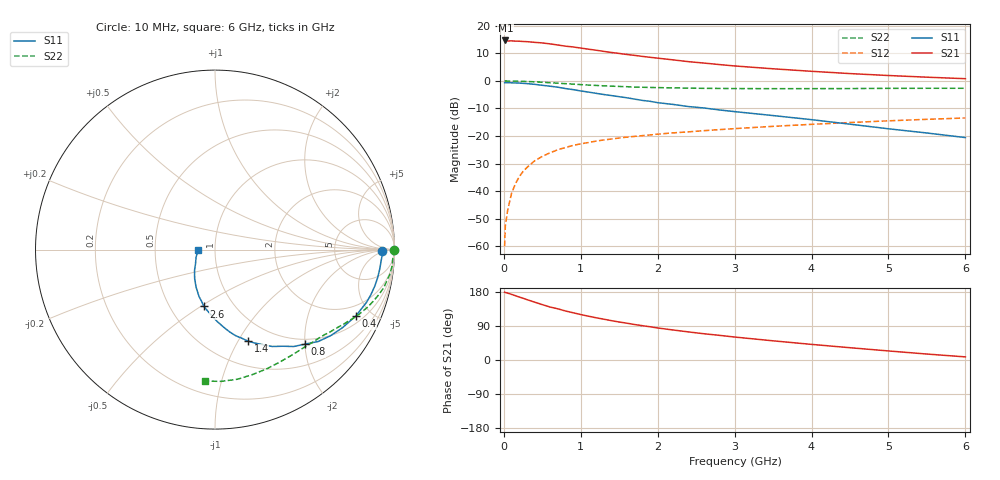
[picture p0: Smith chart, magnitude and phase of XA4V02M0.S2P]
! SIEMENS Discrete & RF Semiconductors
! BFY180
! Si NPN RF Bipolar Junction Transistor in MICRO-X
! VCE = 4 V  IC = 2 mA
! Common Emitter S-Parameters:  May  1997
# GHz  S  MA  R  50
!  f  S11  S21  S12  S22
! GHz  MAG  ANG  MAG  ANG  MAG  ANG  MAG  ANG
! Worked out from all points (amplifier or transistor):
!   36 points, 10 MHz to 6 GHz, reference 50 ohm
!   highest |S21| = 14.7 dB at 20 MHz (marker M1)
!   |S21| within 3 dB of that: start of sweep to 1.059 GHz
!   unconditionally stable (mu >= 1): 2.881 GHz to end of sweep
!   at 250 MHz: K = 0.13, MSG = 23.6 dB, |S12| = -32.9 dB
!   at 1.4 GHz: K = 0.67, MSG = 15.7 dB, |S12| = -21.1 dB
!   at 6 GHz: K = 1.06, MAG = 5.6 dB, |S12| = -13.5 dB
!   S11 on the Smith chart (normalised r, x): 10 MHz: 26, -4; 400 MHz: 1.35, -4.03; 800 MHz: 0.90, -2.00; 1.4 GHz: 0.76, -1.10; 2.6 GHz: 0.73, -0.52; 6 GHz: 0.83, -0.00
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0.01  0.9286 -0.6  5.365 179.0  0.001 88.0  0.9949 -0.2
0.02  0.933 -1.5  5.428 178.1  0.0024 83.0  0.9999 -0.7
0.05  0.9292 -3.1  5.312 176.6  0.0045 87.0  0.9962 -1.6
0.1  0.9242 -6.7  5.341 173.2  0.0091 88.2  0.991 -3.4
0.15  0.9196 -9.8  5.277 169.7  0.0135 84.3  0.9923 -5.0
0.25  0.904 -16.2  5.2 163.0  0.0227 79.3  0.983 -8.3
0.3  0.8938 -19.2  5.159 159.3  0.0268 78.0  0.9756 -9.7
0.4  0.867 -25.3  5.018 152.7  0.0354 74.1  0.964 -12.7
0.5  0.8329 -31.5  4.893 146.1  0.0427 70.8  0.9456 -15.5
0.6  0.8023 -36.8  4.705 139.8  0.0495 67.3  0.9272 -18.1
0.8  0.7271 -46.4  4.279 129.4  0.0618 61.7  0.8918 -22.7
0.9  0.6958 -50.9  4.137 124.7  0.0675 59.3  0.8753 -24.7
1.1  0.6273 -59.4  3.77 115.6  0.0762 55.0  0.8413 -28.4
1.4  0.542 -70.2  3.284 103.8  0.0882 50.8  0.8029 -33.3
1.7  0.4675 -79.7  2.91 93.6  0.0984 47.3  0.7748 -37.5
2  0.4026 -88.0  2.591 84.5  0.1082 44.5  0.7564 -41.6
2.2  0.3744 -92.0  2.411 79.2  0.1139 42.7  0.7476 -44.2
2.6  0.3228 -101.1  2.111 69.3  0.125 39.8  0.7339 -49.2
3.5  0.235 -116.6  1.66 50.6  0.1498 33.8  0.7231 -60.3
4.5  0.1639 -134.2  1.359 32.4  0.1757 26.8  0.7268 -73.3
5.5  0.1134 -158.4  1.169 15.7  0.2009 19.3  0.7349 -87.2
6  0.0936 -178.3  1.098 8.2  0.2125 15.1  0.7348 -94.2
